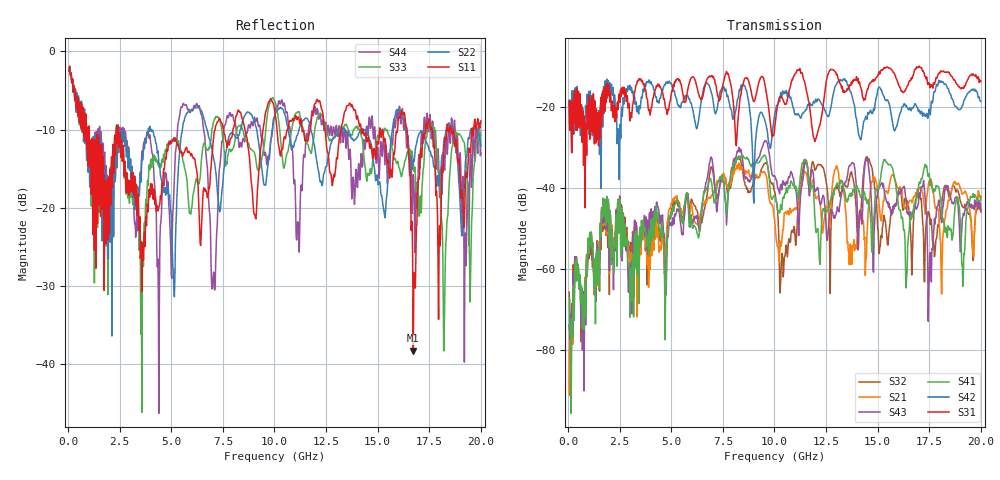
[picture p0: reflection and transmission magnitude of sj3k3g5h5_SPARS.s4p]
! FILE: E:\users\goganessyan\GBX_Backplane\FR408_backplane\1m_OUTBOUND_NEXT\sj3k3g5h5_SPARS.s4p
# MHZ S RI R 50.00
! FREQ  S11  S12  S13  S14
!  S21  S22  S23  S24
!  S31  S32  S33  S34
!  S41  S42  S43  S44
!  REAL  IMAG  REAL  IMAG  REAL  IMAG  REAL  IMAG
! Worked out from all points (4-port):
!   799 points, 50 MHz to 20 GHz, reference 50 ohm
!   strongest paths, dB at 50 MHz, 5.025 GHz, 10.03 GHz, 15.03 GHz, 20 GHz:
!     S31: -18.5, -16.1, -24.2, -12.0, -13.6
!     S42: -18.3, -14.7, -21.3, -15.3, -18.6
!     S41: -66.9, -46.7, -42.0, -40.1, -42.3
!     S43: -73.8, -49.3, -37.1, -40.7, -45.5
!     S21: -90.6, -43.6, -48.9, -41.6, -42.2
!     S32: -65.7, -45.1, -41.1, -50.8, -45.9
!   lowest |S11| = -38.3 dB at 16.73 GHz (marker M1), VSWR 1.02, Z = 50.1 - j1.21 ohm
!   |S11| at or under -10 dB: 1.027 GHz to 2.332 GHz (1.305 GHz wide, 77.7 % of centre); 2.432 GHz to 7.118 GHz (4.686 GHz wide, 98.1 % of centre); 18.56 GHz to 19.56 GHz (1.002 GHz wide, 5.26 % of centre)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
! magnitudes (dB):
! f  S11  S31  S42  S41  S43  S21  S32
! 50 MHz  -2.5  -18.5  -18.3  -66.9  -73.8  -90.6  -65.7
! 3.575 GHz  -30.8  -13.7  -17.8  -49.3  -49.6  -48.4  -51.8
! 8.3 GHz  -7.7  -19.4  -15.6  -32.4  -30.3  -34.9  -32.9
! 10.32 GHz  -12.9  -17.3  -16.9  -44.7  -39.5  -54.3  -59.3
! 11.5 GHz  -11.4  -14.7  -20.6  -33.1  -33.4  -35.9  -32.9
! 16.73 GHz  -38.3  -12.1  -20.1  -46.4  -45.4  -42.3  -49.2
! 20 GHz  -8.9  -13.6  -18.6  -42.3  -45.5  -42.2  -45.9
